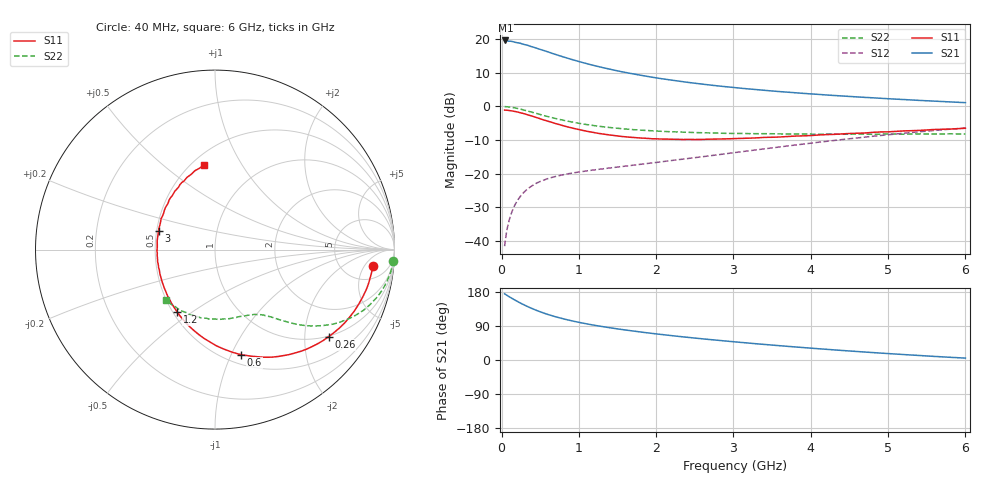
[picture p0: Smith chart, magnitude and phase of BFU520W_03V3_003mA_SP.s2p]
! Filename:  P:\Prog\Test\Noise\ATS_data\Testdata_Net\Run2\BFU520W_APM2013_06_A05_03p3V_003mA_SP_CM01_D.s2p
! Date/Time: Tue 26/Mar/2013 18:01:38
! BFU520W_APM2013_06_A05_03p3V_1to20mA_SP_CM01_Bias3_R.s2p
! MDIF S-parameter v. bias file
! BFU520W_APM2013_06_A05_03p3V_1to20mA_SP_CM01
! Date/time Tue Mar 19 16:47:37 2013
! VAR V_out= 3.3000
! VAR I_out= 2.9950
! VAR V_in= 0.8216
! VAR I_in= 0.0339
! Device data file deembeded for feedlines and parallel
! Original file: \Run2\BFU520W_APM2013_06_A05_03p3V_003mA_SP_CM01_R.s2p
! Feed-files: PR019V01_070313_Feed1.s2p, PR019V01_070313_Feed2.s2p
! Parallel-file: PR019V01_070313_Par.s2p
# MHz S MA R 50
!  Freq-MHz  S11-mag  S11-arg  S21-mag  S21-arg  S12-mag  S12-arg  S22-mag  S22-arg
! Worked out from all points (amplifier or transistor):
!   98 points, 40 MHz to 6 GHz, reference 50 ohm
!   highest |S21| = 19.7 dB at 50 MHz (marker M1)
!   |S21| within 3 dB of that: start of sweep to 547 MHz
!   unconditionally stable (mu >= 1): 2.07 GHz to 3.357 GHz
!   at 300 MHz: K = 0.23, MSG = 21.9 dB, |S12| = -25.4 dB
!   at 1.6 GHz: K = 0.90, MSG = 14.0 dB, |S12| = -17.8 dB
!   at 6 GHz: K = 0.85, MSG = 3.8 dB, |S12| = -6.4 dB
!   S11 on the Smith chart (normalised r, x): 40 MHz: 9, -8; 260 MHz: 0.98, -2.62; 600 MHz: 0.59, -1.09; 1.2 GHz: 0.53, -0.44; 3 GHz: 0.51, +0.12; 6 GHz: 0.57, +0.69
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40  0.8839 -6.1  9.619 174.7  0.00828 85.8  0.9945 -3.5
50  0.8829 -7.6  9.636 173.4  0.01029 85.2  0.9942 -4.4
140  0.8561 -21.0  9.288 162.0  0.02794 77.9  0.9659 -12.2
220  0.8194 -32.2  8.871 152.9  0.0419 72.0  0.9257 -18.2
260  0.7978 -37.5  8.618 148.7  0.04824 69.3  0.9038 -21.0
320  0.7625 -45.4  8.272 142.6  0.05669 65.7  0.8664 -24.9
420  0.7026 -57.2  7.611 133.6  0.06854 60.8  0.8056 -30.1
500  0.6562 -66.0  7.093 127.3  0.07623 57.6  0.7594 -33.5
600  0.6035 -76.0  6.522 120.2  0.08411 54.6  0.7063 -37.0
700  0.5561 -85.0  5.966 114.0  0.09058 52.4  0.6613 -39.9
800  0.5156 -93.1  5.475 108.7  0.09618 51.0  0.623 -42.1
900  0.4818 -100.8  5.053 103.8  0.1011 50.0  0.5906 -43.9
1050  0.4406 -111.2  4.512 97.4  0.1073 49.3  0.549 -46.2
1200  0.4074 -120.9  4.07 91.8  0.1134 49.1  0.5181 -48.2
1550  0.3577 -140.7  3.304 80.6  0.127 50.0  0.4672 -52.2
2050  0.3277 -164.1  2.616 67.8  0.1489 52.8  0.4276 -57.7
2500  0.3219 177.8  2.222 57.9  0.1726 54.8  0.4087 -63.6
3000  0.3318 161.4  1.92 48.2  0.2044 56.4  0.3965 -71.2
3100  0.3345 158.3  1.869 46.4  0.2112 56.5  0.3962 -72.7
4100  0.3759 133.0  1.514 29.7  0.293 54.8  0.3863 -91.0
5200  0.4321 111.1  1.269 14.4  0.3991 47.6  0.3858 -114.6
6000  0.4734 97.7  1.14 5.0  0.4778 40.2  0.3891 -134.1
